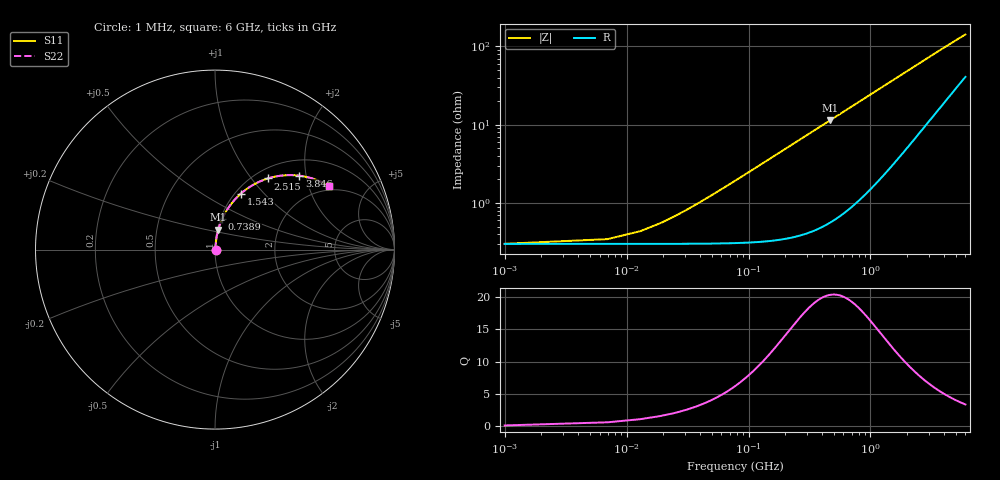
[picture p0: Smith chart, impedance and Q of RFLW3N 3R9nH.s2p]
!Vishay Electro-Films
!RFLW3N3900C - 3.9 nH Spiral Inductor on Quartz
!Measured in series configuration
!May 2011
# GHz S MA R 50
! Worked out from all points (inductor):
!   1001 points, 1 MHz to 6 GHz, reference 50 ohm
!   read as one part in series: L = 3.9 nH near 36.99 MHz
!   highest Q = 20.4 at 468.9 MHz (marker M1), where L = 3.89 nH
!   S11 on the Smith chart (normalised r, x): 1 MHz: 1.01, +0.00; 738.9 MHz: 1.02, +0.36; 1.543 GHz: 1.06, +0.75; 2.515 GHz: 1.16, +1.21; 3.846 GHz: 1.35, +1.83; 6 GHz: 1.82, +2.73
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0.001  0.002999 4.7  0.997 -0.0  0.997 -0.0  0.002999 4.7
0.018997  0.005518 56.9  0.997 -0.3  0.997 -0.3  0.005518 56.9
0.048992  0.01233 75.1  0.9969 -0.7  0.9969 -0.7  0.01233 75.1
0.066989  0.01662 78.5  0.9968 -0.9  0.9968 -0.9  0.01662 78.5
0.096984  0.02386 81.2  0.9966 -1.4  0.9966 -1.4  0.02386 81.2
0.138977  0.03404 82.6  0.9962 -1.9  0.9962 -1.9  0.03404 82.6
0.198967  0.04859 83.1  0.9954 -2.8  0.9954 -2.8  0.04859 83.1
0.270955  0.06602 82.9  0.994 -3.8  0.994 -3.8  0.06602 82.9
0.36094  0.08769 82.0  0.9916 -5.0  0.9916 -5.0  0.08769 82.0
0.468922  0.1135 80.7  0.988 -6.5  0.988 -6.5  0.1135 80.7
0.594901  0.1431 78.9  0.9826 -8.2  0.9826 -8.2  0.1431 78.9
0.738877  0.1764 76.8  0.9751 -10.1  0.9751 -10.1  0.1764 76.8
1.00283  0.235 72.9  0.9577 -13.6  0.9577 -13.6  0.235 72.9
1.25479  0.2877 69.2  0.9375 -16.7  0.9375 -16.7  0.2877 69.2
1.54274  0.3435 65.2  0.911 -20.0  0.911 -20.0  0.3435 65.2
2.00467  0.4224 59.2  0.8636 -24.8  0.8636 -24.8  0.4224 59.2
2.51458  0.4949 53.3  0.8082 -29.4  0.8082 -29.4  0.4949 53.3
3.0005  0.5511 48.4  0.756 -33.0  0.756 -33.0  0.5511 48.4
3.84636  0.6246 41.3  0.6717 -37.8  0.6717 -37.8  0.6246 41.3
4.00233  0.6354 40.1  0.6575 -38.5  0.6575 -38.5  0.6354 40.1
5.00417  0.6901 33.9  0.5756 -42.0  0.5756 -42.0  0.6901 33.9
6  0.7263 29.2  0.5099 -44.1  0.5099 -44.1  0.7263 29.2
